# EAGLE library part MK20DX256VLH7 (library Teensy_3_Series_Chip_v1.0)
This is a footprint for the MK20dx256VHL7, the chip at the heart of the Teensy 3.1. Notable upgrades over the Teensy 3.0 include more Flash Memory, RAM, a DAC output, additional ADC pins, etc. Remember, if you want to use USB, VOut3v3 has to be attached to the 3.3V bus.
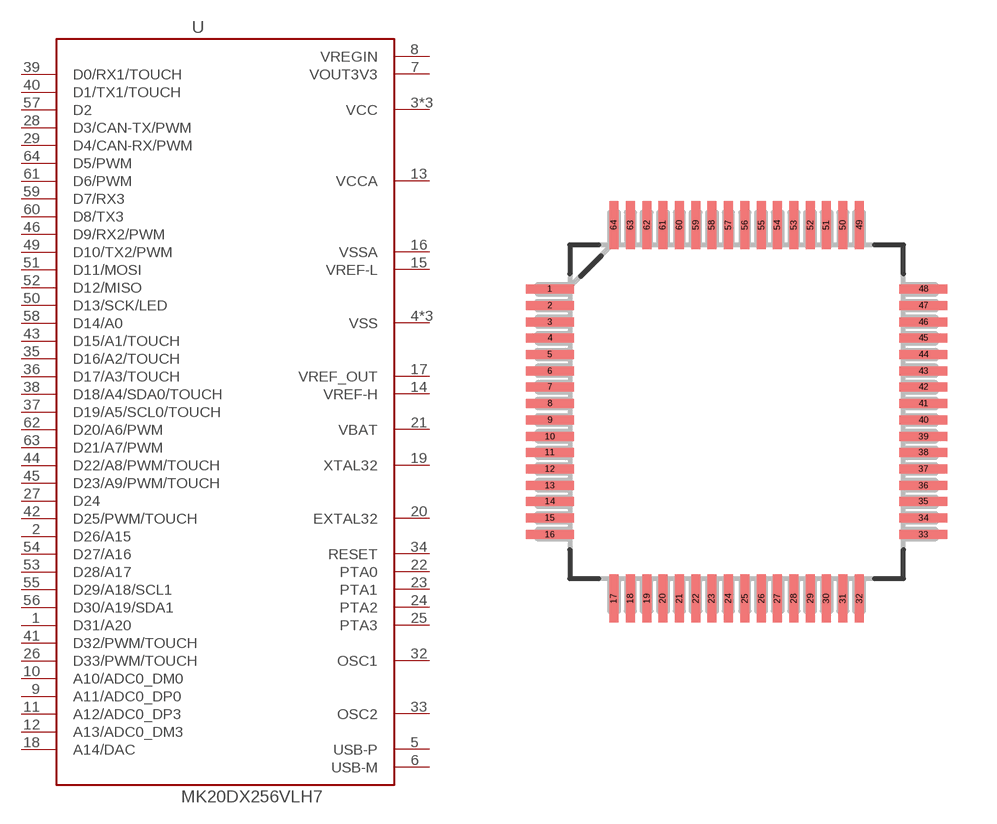
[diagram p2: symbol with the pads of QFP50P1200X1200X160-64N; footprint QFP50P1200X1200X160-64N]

Designator prefix -

## MK20DX256VLH7  [QFP50P1200X1200X160-64N]
1  D31/A20
2  D26/A15
3  VCC
4  VSS
5  USB-P
6  USB-M
7  VOUT3V3
8  VREGIN
9  A11/ADC0_DP0
10  A10/ADC0_DM0
11  A12/ADC0_DP3
12  A13/ADC0_DM3
13  VCCA
14  VREF-H
15  VREF-L
16  VSSA
17  VREF_OUT
18  A14/DAC
19  XTAL32
20  EXTAL32
21  VBAT
22  PTA0
23  PTA1
24  PTA2
25  PTA3
26  D33/PWM/TOUCH
27  D24
28  D3/CAN-TX/PWM
29  D4/CAN-RX/PWM
30  VCC
31  VSS
32  OSC1
33  OSC2
34  RESET
35  D16/A2/TOUCH
36  D17/A3/TOUCH
37  D19/A5/SCL0/TOUCH
38  D18/A4/SDA0/TOUCH
39  D0/RX1/TOUCH
40  D1/TX1/TOUCH
41  D32/PWM/TOUCH
42  D25/PWM/TOUCH
43  D15/A1/TOUCH
44  D22/A8/PWM/TOUCH
45  D23/A9/PWM/TOUCH
46  D9/RX2/PWM
47  VSS
48  VCC
49  D10/TX2/PWM
50  D13/SCK/LED
51  D11/MOSI
52  D12/MISO
53  D28/A17
54  D27/A16
55  D29/A18/SCL1
56  D30/A19/SDA1
57  D2
58  D14/A0
59  D7/RX3
60  D8/TX3
61  D6/PWM
62  D20/A6/PWM
63  D21/A7/PWM
64  D5/PWM

## Footprint QFP50P1200X1200X160-64N (pad centres in mm)
smd 1.473 x 0.279: 1 -5.715,3.759; 2 -5.715,3.251; 3 -5.715,2.743; 4 -5.715,2.261; 5 -5.715,1.753; 6 -5.715,1.245; 7 -5.715,0.762; 8 -5.715,0.254; 9 -5.715,-0.254; 10 -5.715,-0.762; 11 -5.715,-1.245; 12 -5.715,-1.753; 13 -5.715,-2.261; 14 -5.715,-2.743; 15 -5.715,-3.251; 16 -5.715,-3.759; 33 5.715,-3.759; 34 5.715,-3.251; 35 5.715,-2.743; 36 5.715,-2.261; 37 5.715,-1.753; 38 5.715,-1.245; 39 5.715,-0.762; 40 5.715,-0.254; 41 5.715,0.254; 42 5.715,0.762; 43 5.715,1.245; 44 5.715,1.753; 45 5.715,2.261; 46 5.715,2.743; 47 5.715,3.251; 48 5.715,3.759
smd 0.279 x 1.473: 17 -3.759,-5.715; 18 -3.251,-5.715; 19 -2.743,-5.715; 20 -2.261,-5.715; 21 -1.753,-5.715; 22 -1.245,-5.715; 23 -0.762,-5.715; 24 -0.254,-5.715; 25 0.254,-5.715; 26 0.762,-5.715; 27 1.245,-5.715; 28 1.753,-5.715; 29 2.261,-5.715; 30 2.743,-5.715; 31 3.251,-5.715; 32 3.759,-5.715; 49 3.759,5.715; 50 3.251,5.715; 51 2.743,5.715; 52 2.261,5.715; 53 1.753,5.715; 54 1.245,5.715; 55 0.762,5.715; 56 0.254,5.715; 57 -0.254,5.715; 58 -0.762,5.715; 59 -1.245,5.715; 60 -1.753,5.715; 61 -2.261,5.715; 62 -2.743,5.715; 63 -3.251,5.715; 64 -3.759,5.715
